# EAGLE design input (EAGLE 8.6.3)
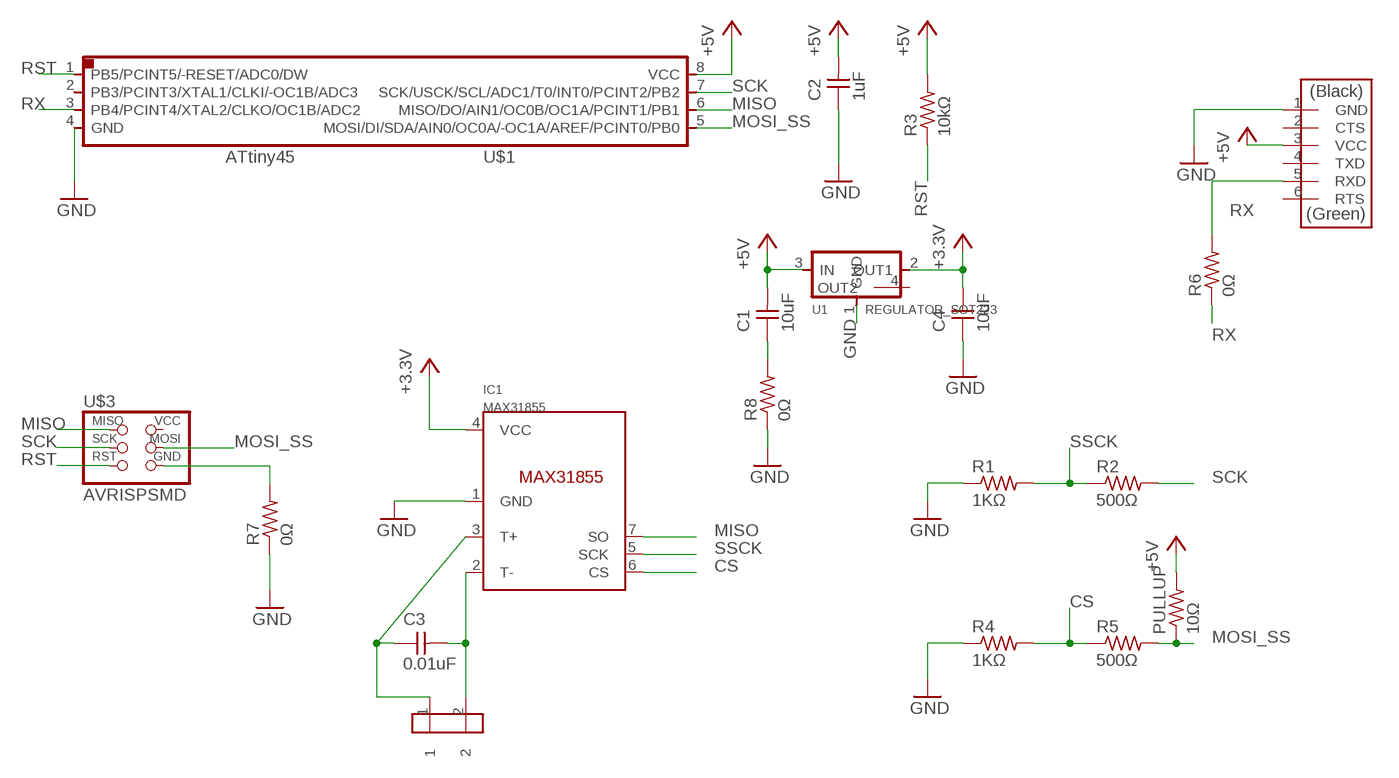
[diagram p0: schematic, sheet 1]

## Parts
C1  10uF  CAP-UNPOLARIZEDFAB  [C1206FAB]
C2  1uF  CAP-UNPOLARIZED  [C1206]
C3  0.01uF  CAP-UNPOLARIZEDFAB  [C1206FAB]
C4  10uF  CAP-UNPOLARIZEDFAB  [C1206FAB]
IC1  MAX31855  [SOIC8]
PULLUP  10Ω  RES-US1206FAB  [R1206FAB]
R1  1KΩ  RES-US1206FAB  [R1206FAB]
R2  500Ω  RES-US1206FAB  [R1206FAB]
R3  10kΩ  RES-US1206  [R1206]
R4  1KΩ  RES-US1206FAB  [R1206FAB]
R5  500Ω  RES-US1206FAB  [R1206FAB]
R6  0Ω  RES-US1206FAB  [R1206FAB]
R7  0Ω  RES-US1206FAB  [R1206FAB]
R8  0Ω  RES-US1206FAB  [R1206FAB]
TML1  AKIZUKITNK_HOLE2PIN  [5.08PICH_HL]
U1  REGULATOR_SOT223  [SOT223]
U$1  ATTINY45SI  [SOIC8]
U$2  FTDI-SMD-HEADER  [1X06SMD]
U$3  AVRISPSMD  [2X03SMD]

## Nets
3.3V: C4.2 IC1.4(VCC) U1.2(OUT1) ; supply symbol labelled +3.3V
+5V: C1.2 C2.2 PULLUP.2 R3.2 U1.3(IN) U$1.8(VCC) U$2.3(VCC)
CS: IC1.6(CS) R4.2 R5.1
GND: C1.1 C2.1 C4.1 IC1.1(GND) R1.1 R4.1 R7.1 R7.2 R8.1 R8.2 U1.1(GND) U$1.4(GND) U$2.1(GND) U$3.6(GND)
MISO: IC1.7(SO) U$1.6(MISO/DO/AIN1/OC0B/OC1A/PCINT1/PB1) U$3.1(MISO)
MOSI_SS: PULLUP.1 R5.2 U$1.5(MOSI/DI/SDA/AIN0/OC0A/-OC1A/AREF/PCINT0/PB0) U$3.4(MOSI)
N$2: C3.1 IC1.3(T+) TML1.1
N$3: C3.2 IC1.2(T-) TML1.2
RST: R3.1 U$1.1(PB5/PCINT5/-RESET/ADC0/DW) U$3.5(RST)
RX: R6.1 R6.2 U$1.3(PB4/PCINT4/XTAL2/CLKO/OC1B/ADC2) U$2.5(RXD)
SCK: R2.2 U$1.7(SCK/USCK/SCL/ADC1/T0/INT0/PCINT2/PB2) U$3.3(SCK)
SSCK: IC1.5(SCK) R1.2 R2.1
Unconnected: U1.4(OUT2) U$1.2(PB3/PCINT3/XTAL1/CLKI/-OC1B/ADC3) U$2.2(CTS) U$2.4(TXD) U$2.6(RTS) U$3.2(VCC)

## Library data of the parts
C1-C4 = fab:CAP-UNPOLARIZED
IC1 = AlexW-Eagle-Libraries 2:MAX31855
PULLUP R1 R2 R4-R8 = fab:RES-US: Resistor (US Symbol)
R3 = HelloKamakura:RES-US: Resistor (US Symbol)
TML1 = doyo:AKIZUKI?TNK_HOLE2PIN
U1 = fab:REGULATOR_SOT223
U$1 = fab:ATTINY45
U$2 = fab:FTDI-SMD-HEADER
U$3 = HelloKamakura:AVRISP

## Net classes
0 default: width 0.406 mm

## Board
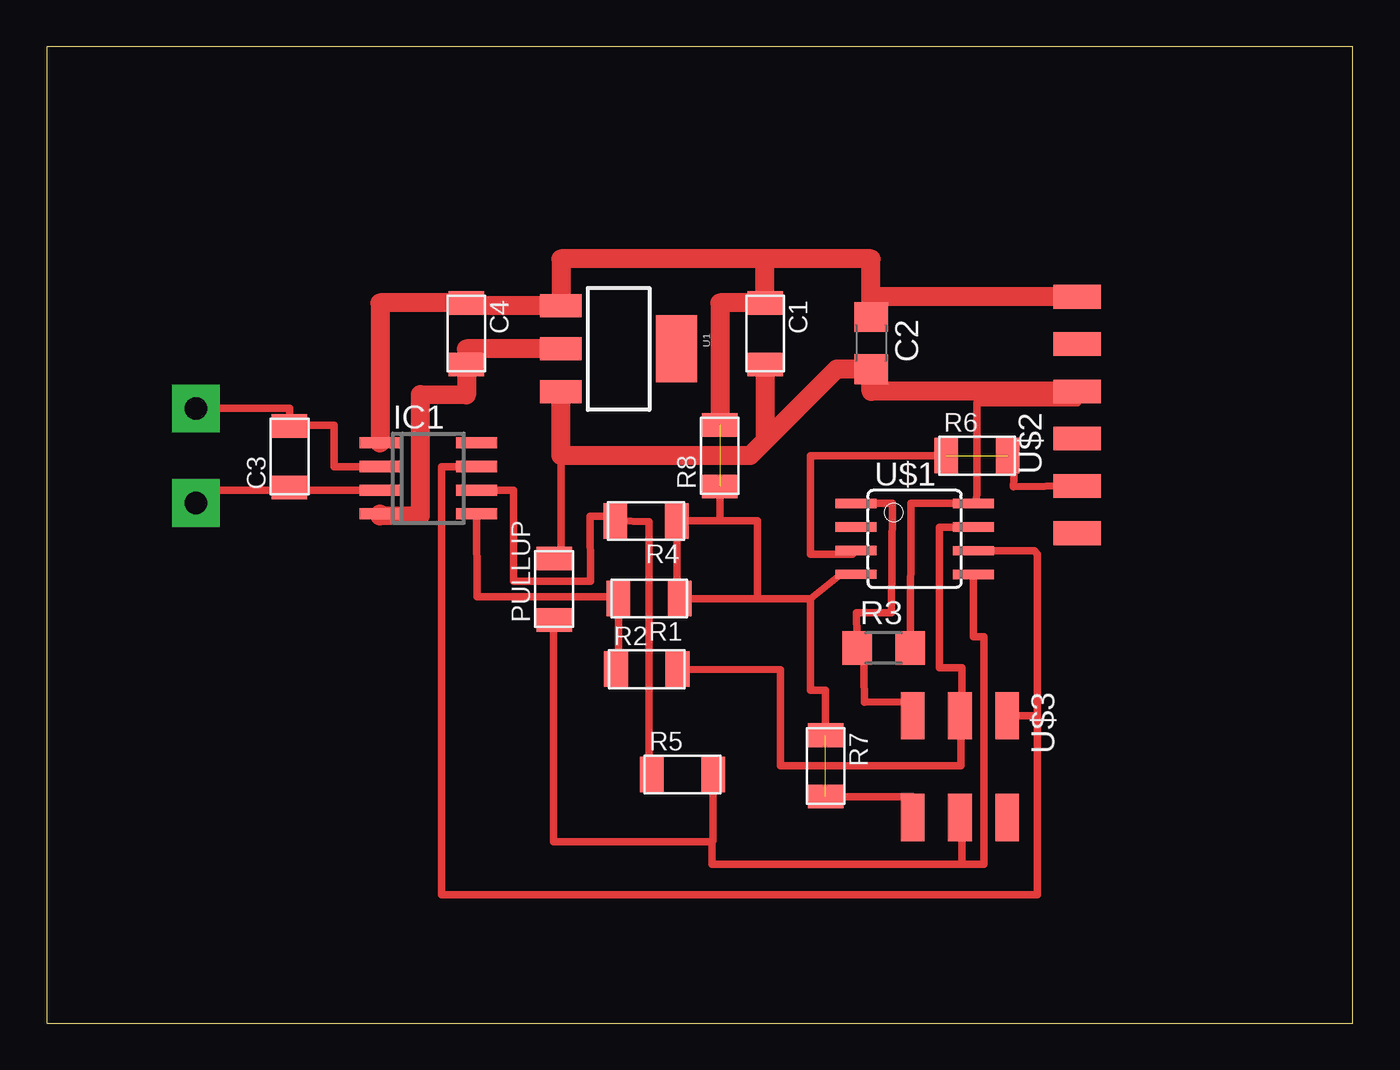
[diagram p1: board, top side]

Size 70.19 x 52.45 mm. Coordinates in mm from the lower left corner, seen from the top.
Outline: 0,0 70.19,0 70.19,52.45 0,52.45 0,0
Copper layers (1*16): Top 0.035mm / dielectric 1.5mm / Bottom 0.035mm
Design rules "default *": minimum track width 6mil, minimum drill 0.35mm, track to track 0.4mm, track to pad 0.4mm, pad to pad 0.4mm, via to via 0.4mm, smd to smd 0.4mm, copper to edge 40mil, drill to drill 6mil, minimum pad ring 10mil, minimum via ring 8mil, stop-mask expansion 4mil, vias tented up to drill 0mil, thermal gap 10mil

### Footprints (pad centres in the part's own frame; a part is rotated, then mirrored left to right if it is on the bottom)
C1206FAB = smd 1.27 x 1.905: 1 -1.651,0; 2 1.651,0
C1206 = smd 1.6 x 1.8: 1 -1.4,0; 2 1.4,0
SOIC8 = smd 0.6 x 2.2: 1 -1.905,-2.6; 2 -0.635,-2.6; 3 0.635,-2.6; 4 1.905,-2.6; 5 1.905,2.6; 6 0.635,2.6; 7 -0.635,2.6; 8 -1.905,2.6
R1206FAB = smd 1.27 x 1.905: 1 -1.651,0; 2 1.651,0
R1206 = smd 1.6 x 1.803: 1 -1.422,0; 2 1.422,0
5.08PICH_HL = drill 1.2 pad 2.54 square: 1 0,0; 2 -5.08,0
SOT223 = smd 1.219 x 2.235: 1 -2.311,-3.099; 2 0,-3.099; 3 2.311,-3.099 | smd 3.6 x 2.2: 4 0,3.099
SOIC8' = smd 0.5 x 2.2: 1 -1.905,-3.154; 2 -0.645,-3.154; 3 0.625,-3.154; 4 1.895,-3.154; 5 1.905,3.154; 6 0.635,3.154; 7 -0.635,3.154; 8 -1.905,3.154
1X06SMD = smd 2.54 x 1.27: 1 0,6.35; 2 0,3.81; 3 0,1.27; 4 0,-1.27; 5 0,-3.81; 6 0,-6.35
2X03SMD = smd 2.54 x 1.27: 1 -2.54,2.54; 2 2.92,2.54; 3 -2.54,0; 4 2.92,0; 5 -2.54,-2.54; 6 2.92,-2.54

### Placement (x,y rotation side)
C1  38.61,37.03 270 top
C2  44.3,36.53 270 top
C3  13.06,30.43 90 top
C4  22.56,37.03 270 top
IC1  20.51,29.26 270 top
PULLUP  27.27,23.31 90 top
R1  32.37,22.81 180 top
R2  32.25,19.01 0 top
R3  44.98,20.15 0 top
R4  32.21,26.97 180 top
R5  34.16,13.36 0 top
R6  49.99,30.48 0 top
R7  41.86,13.82 270 top
R8  36.17,30.48 90 top
TML1  8.03,27.94 270 top
U1  30.73,36.22 270 top
U$1  ATTINY45SI  [SOIC8']  46.63,26.01 270 top
U$2  55.37,32.66 0 top
U$3  49.07,13.97 270 top

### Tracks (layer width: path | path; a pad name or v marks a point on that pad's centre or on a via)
3.3V
  Top 1.016: U1.2 22.55,36.22 C4.2 22.55,33.73 20.07,33.76 20.07,27.25 17.91,27.23 IC1.4
+5V
  Top 0.406: U$2.3 55.37,33.33 49.99,33.33 49.99,28.52 49.95,28.08 49.95,27.91 U$1.8 46.43,27.91 R3.2 | PULLUP.2 27.64,24.97 27.64,30.89
  Top 1.016: U$2.3 44.3,33.93 C2.2 42.44,35.12 38.61,31.29 | 38.61,31.29 37.8,30.48 27.64,30.48 27.64,30.89 U1.3 | C1.2 38.61,31.29
CS
  Top 0.406: R5.1 32.36,13.33 32.36,26.94 R4.2 30.56,27.23 29.21,27.23 29.21,23.72 25.09,23.72 25.08,28.63 IC1.6
GND  (2 unrouted)
  Top 0.406: 35.89,22.81 R1.1 | 41.05,22.81 38.2,22.81 | 38.2,22.81 R1.1 | U$1.4 42.67,24.11 41.05,22.81 | 38.2,22.81 38.2,26.98 36.17,26.98 | 36.17,26.98 R4.1 33.86,22.81 R1.1 | R7.2 46.53,12.17 U$3.6 | 41.05,22.81 41.05,17.88 41.86,17.88 R7.1 | 36.17,26.98 R8.1
  Top 1.016: U$2.1 44.3,39.01 C2.1 44.3,41.05 38.61,41.05 | 38.61,41.05 27.64,41.05 U1.1 22.55,38.53 C4.1 17.91,38.68 IC1.1 | 38.61,41.05 C1.1 36.17,38.68 R8.2
MISO
  Top 0.406: U$1.6 53.06,25.38 53.24,25.2 53.24,16.26 | 53.24,16.26 52.98,16.51 U$3.1 | 53.24,16.26 53.24,6.91 21.23,6.91 21.23,29.9 IC1.7
MOSI_SS
  Top 0.406: R5.2 35.81,9.8 | 35.81,9.8 35.76,9.75 27.23,9.75 27.23,21.62 PULLUP.1 | 35.81,9.8 35.76,9.8 35.76,8.53 49.17,8.53 | U$3.4 49.17,11.05 49.17,8.53 | U$1.5 49.79,20.77 50.37,20.77 50.37,8.53 49.17,8.53
N$2
  Top 0.406: IC1.3 13.87,28.63 | 13.87,28.63 C3.1 | TML1.1 8.84,28.63 13.87,28.63
N$3
  Top 0.406: IC1.2 15.44,29.9 15.44,32.11 13.06,32.11 C3.2 13.06,33.02 TML1.2
RST
  Top 0.406: 43.9,20.33 R3.1 43.54,20.73 43.51,22.03 45.4,22.03 45.43,27.91 U$1.1 | 43.9,20.33 43.95,17.24 46.53,17.27 U$3.5 | 43.48,20.74 43.9,20.33
RX  (1 unrouted)
  Top 0.406: R6.1 41.05,30.48 41.05,25.2 43.29,25.2 U$1.3 | R6.2 52.02,30.1 51.96,28.82 U$2.5
SCK
  Top 0.406: R2.2 39.42,18.99 39.42,13.82 49.14,13.82 49.14,16.26 | 49.14,16.26 49.14,16.51 U$3.3 | U$1.7 47.95,26.64 47.95,19.1 49.17,19.1 49.17,16.26 49.14,16.26
SSCK
  Top 0.406: IC1.5 23.14,22.9 30.75,22.9 R1.2 30.72,19.01 R2.1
